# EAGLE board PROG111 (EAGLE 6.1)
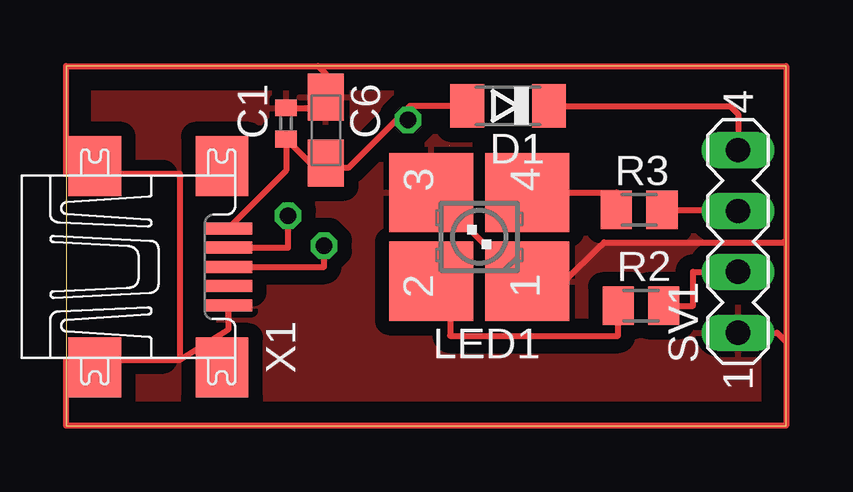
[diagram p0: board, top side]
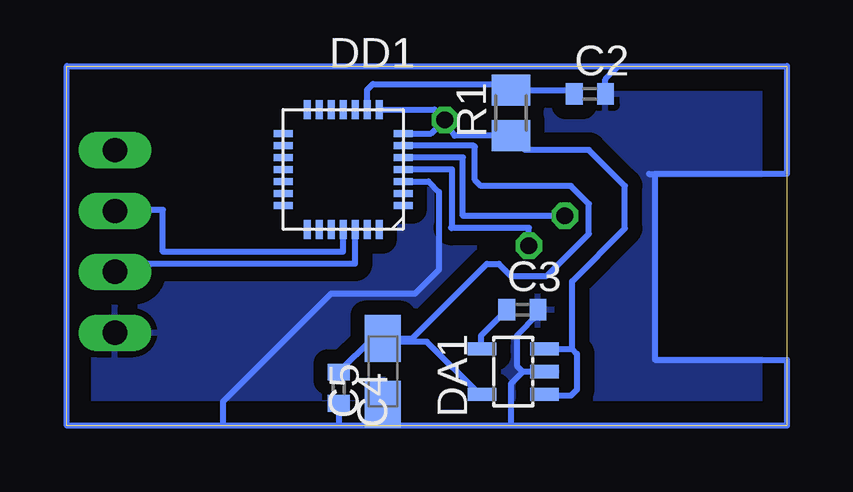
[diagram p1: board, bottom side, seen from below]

Size 30 x 15 mm. Coordinates in mm from the lower left corner, seen from the top.
Outline: 0,0 30,0 30,15 0,15 0,0
Copper layers (1*16): Top 0.035mm / dielectric 1.5mm / Bottom 0.035mm
Design rules: minimum track width 10mil, minimum drill 24mil, track to track 8mil, track to pad 8mil, pad to pad 8mil, via to via 8mil, smd to smd 8mil, copper to edge 40mil, drill to drill 8mil, minimum pad ring 10mil, minimum via ring 8mil, stop-mask expansion 4mil, vias tented up to drill 0mil, thermal gap 10mil

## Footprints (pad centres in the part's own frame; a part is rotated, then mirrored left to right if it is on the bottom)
C0402 = smd 0.7 x 0.9: 1 -0.65,0; 2 0.65,0
A/3216-18R = smd 1.95 x 1.5: + 1.375,0; - -1.375,0
SOD80C = smd 1.4 x 1.8: A 1.7,0; C -1.7,0
SOT23-5L = smd 0.55 x 1.2: 1 -0.95,-1.3; 2 0,-1.3; 3 0.95,-1.3; 4 0.95,1.3; 5 -0.95,1.3
QFN-28 = smd 0.8 x 0.3: 1 -2.5,1.5; 2 -2.5,1; 3 -2.5,0.5; 4 -2.5,0; 5 -2.5,-0.5; 6 -2.5,-1; 7 -2.5,-1.5; 15 2.5,-1.5; 16 2.5,-1; 17 2.5,-0.5; 18 2.5,0; 19 2.5,0.5; 20 2.5,1; 21 2.5,1.5 | smd 0.3 x 0.8: 8 -1.5,-2.5; 9 -1,-2.5; 10 -0.5,-2.5; 11 0,-2.5; 12 0.5,-2.5; 13 1,-2.5; 14 1.5,-2.5; 22 1.5,2.5; 23 1,2.5; 24 0.5,2.5; 25 0,2.5; 26 -0.5,2.5; 27 -1,2.5; 28 -1.5,2.5
P-LCC-4/2 = smd 3.3 x 3.5: 1 -1.85,-2; 2 -1.85,2; 3 1.85,2; 4 1.85,-2
M2012 = smd 1.3 x 1.6: 1 -0.95,0; 2 0.95,0
MA04-1 = drill 1.016 long: 1 -3.81,0; 2 -1.27,0; 3 1.27,0; 4 3.81,0
UX60A-MB-5ST = smd 2 x 0.5: 1 2.25,1.6; 2 2.25,0.8; 3 2.25,0; 4 2.25,-0.8; 5 2.25,-1.6 | smd 2.2 x 2.5: M1 -3.3,-4.2; M2 -3.3,4.2; M3 2,4.2; M4 2,-4.2

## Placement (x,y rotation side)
C1  [C0402]  9.17,12.6 90 top
C2  [C0402]  8.21,13.83 0 bottom
C3  [C0402]  11.02,4.83 0 bottom
C4  [C0402]  18.67,1.58 270 bottom
C5  [A/3216-18R]  16.83,2.26 90 bottom
C6  [A/3216-18R]  10.83,12.32 270 top
D1  PMLL41SOD80C  [SOD80C]  18.42,13.33 180 top
DA1  [SOT23-5L]  11.4,2.25 90 bottom
DD1  [QFN-28]  18.49,10.68 180 bottom
LED1  [P-LCC-4/2]  17.22,7.87 90 top
R1  [M2012]  11.5,13.04 90 bottom
R2  [M2012]  23.96,5 0 top
R3  [M2012]  23.88,9 0 top
SV1  [MA04-1]  28,7.68 90 top
X1  MINI-USB-UX60A-MB-5ST  [UX60A-MB-5ST]  4.5,6.62 0 top

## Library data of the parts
C1-C6 R1-R3 = resistor
D1 = diode
DA1 DD1 = pepelac
LED1 = led
SV1 = con-lstb; OC_FARNELL: unknown; OC_NEWARK: unknown
X1 = con-hirose; OC_FARNELL: unknown; OC_NEWARK: unknown

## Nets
GND: C1.2 C2.2 C3.2 C4.2 C5.- C6.- DA1.2 DD1.3 LED1.1 LED1.3 SV1.1 X1.5
N$1: D1.C SV1.4
N$2: DD1.26 R2.2 SV1.2
N$3: DD1.25 R3.2 SV1.3
N$4: C1.1 C6.+ D1.A DA1.1 DA1.3 DD1.7 DD1.8 R1.1 X1.1
N$5: C3.1 DA1.4
N$6: C4.1 C5.+ DA1.5 DD1.6
N$7: C2.1 DD1.9 R1.2
N$8: DD1.5 X1.2
N$9: DD1.4 X1.3
N$10: LED1.2 R2.1
N$11: LED1.4 R3.1

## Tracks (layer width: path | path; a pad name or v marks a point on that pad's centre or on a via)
GND
  Top 0.25: 4.75,2.75 0,2.75 0,0 30,0 30,3.5 | 4.75,2.75 4.75,10.5 0,10.5 0,15 10.5,15 | 10.5,15 30,15 30,7.75 | 30,7.75 30,3.5 | LED1.3 15.28,9.72 17.75,7.25 17.99,7.25 LED1.1 20.77,6.02 22.25,7.5 22.28,7.5 22.42,7.64 29.89,7.64 30,7.75 | SV1.1 29.63,3.87 30,3.5 | 10.5,15 10.83,14.67 C6.- 10.38,13.25 C1.2 | X1.5 6.75,4 4.75,2.75
  Bottom 0.25: 5.75,10.5 5.5,10.5 | 5.5,10.5 0,10.5 0,15 7,15 | 5.5,10.5 5.5,2.75 0,2.75 0,0 11.5,0 | 11.5,0 17,0 | 17,0 18.75,0 | 18.75,0 23.5,0 | 23.5,0 30,0 30,15 7,15 | C2.2 7.56,14.44 7,15 | DA1.2 11,2.25 | 11,2.25 11.5,1.75 11.5,0 | C3.2 10.37,4.63 11.25,3.75 11.25,2.5 11,2.25 | C4.2 18.67,0.08 18.75,0 | C5.- 16.83,0.17 17,0 | DD1.3 14.93,10.18 14.5,9.75 14.5,6.5 15.5,5.5 19,5.5 23.5,1 23.5,0
  pour Top (isolate 0.6): 0,15 30,15 30,0 0,0 0,2.75 4.75,2.75 4.75,10.5 0,10.5
  pour Bottom (isolate 0.6): 0,15 30,15 30,0 0,0 0,2.75 5.5,2.75 5.5,10.5 0,10.5
N$1
  Top 0.25: D1.C 27.67,13.33 28,13 SV1.4
N$2
  Top 0.25: R2.2 26.13,5 26.13,6.41 SV1.2
  Bottom 0.25: DD1.26 18,6.75 28,6.75 SV1.2
N$3
  Top 0.25: R3.2 28,9 SV1.3
  Bottom 0.25: DD1.25 18.5,7.25 26,7.25 26,9 28,9 SV1.3
N$4  (via drill 0.7)
  Top 0.25: D1.A 14.33,13.33 14,13 | 14,13 11.75,10.75 11.03,10.75 C6.+ 10.18,10.95 C1.1 9.17,10.64 X1.1 | v14.25,12.75 14,13
  Bottom 0.25: v14.25,12.75 13.84,12.09 R1.1 10.91,11.5 8.25,11.5 6.75,10 X1.1 8.95,6.02 8.95,3.2 | DA1.3 8.95,3.2 | 8.95,3.2 8.75,3 8.75,1.5 9,1.25 10.05,1.25 DA1.1 | DD1.7 14.82,12.18 v14.25,12.75 | DD1.8 14.68,13.18 v14.25,12.75
N$5
  Bottom 0.25: C3.1 12.75,3.75 12.75,3.25 DA1.4
N$6  (1 unrouted)
  Bottom 0.25: DA1.5 12.8,1.3 15,3.5 16.7,3.5 C5.+ | C5.+ 17.27,3.63 C4.1 | C5.+ 15.62,3.63 12.5,6.75 12,6.75 11.5,6.25 10,6.25 8.25,8 8.25,9.25 9,10 12.75,10 13,10.25 13,11.63 13.04,11.68 DD1.6 16,11.67 16,11.75
N$7
  Bottom 0.25: DD1.9 17.49,14.01 17.25,14.25 12.26,14.25 R1.2 8.95,13.99 C2.1
N$8  (via drill 0.7)
  Top 0.25: X1.2 9.25,7.42 v9.25,8.75
  Bottom 0.25: v9.25,8.75 13.5,8.75 13.5,11.19 DD1.5
N$9  (via drill 0.7)
  Top 0.25: X1.3 10.75,6.62 v10.75,7.5
  Bottom 0.25: v10.75,7.5 10.75,8.25 13.95,8.25 | 14,8.25 13.95,8.25 | 13.95,8.25 13.95,10.68 DD1.4
N$10
  Top 0.25: LED1.2 16,6.02 16,3.75 23.01,3.75 R2.1
N$11
  Top 0.25: LED1.4 22.93,9.72 R3.1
